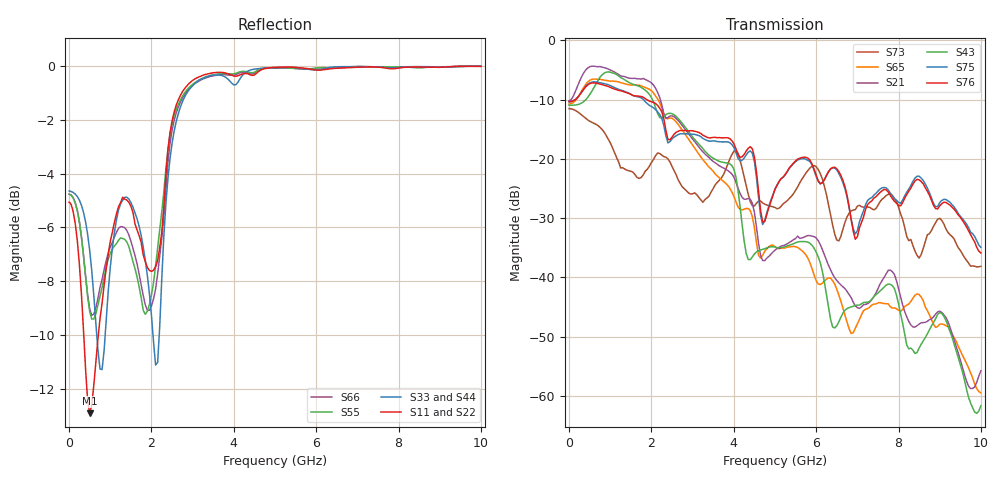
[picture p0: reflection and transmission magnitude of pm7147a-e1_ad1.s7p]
# GHz S DB R 50
! S-Parameters data
! Freq  dbS11  angS11  dbS12  angS12  dbS13  angS13  dbS14  angS14
!  dbS15  angS15  dbS16  angS16  dbS17  angS17  dbS21  angS21
!  dbS22  angS22  dbS23  angS23  dbS24  angS24  dbS25  angS25
!  dbS26  angS26  dbS27  angS27  dbS31  angS31  dbS32  angS32
!  dbS33  angS33  dbS34  angS34  dbS35  angS35  dbS36  angS36
!  dbS37  angS37  dbS41  angS41  dbS42  angS42  dbS43  angS43
!  dbS44  angS44  dbS45  angS45  dbS46  angS46  dbS47  angS47
!  dbS51  angS51  dbS52  angS52  dbS53  angS53  dbS54  angS54
!  dbS55  angS55  dbS56  angS56  dbS57  angS57  dbS61  angS61
!  dbS62  angS62  dbS63  angS63  dbS64  angS64  dbS65  angS65
!  dbS66  angS66  dbS67  angS67  dbS71  angS71  dbS72  angS72
!  dbS73  angS73  dbS74  angS74  dbS75  angS75  dbS76  angS76
!  dbS77  angS77
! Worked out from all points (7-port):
!   279 points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, 1 Hz to 10 GHz, reference 50 ohm
!   strongest paths, dB at 1 Hz, 7.943 MHz, 3.05 GHz, 6.55 GHz, 10 GHz:
!     S76: -10.3, -10.3, -15.3, -22.2, -35.9
!     S75: -10.3, -10.3, -15.9, -22.5, -34.9
!     S43: -10.9, -10.9, -16.7, -47.5, -61.7
!     S21: -10.2, -10.2, -17.1, -40.9, -55.8
!     S65: -10.7, -10.7, -18.2, -43.0, -59.5
!     S73: -11.5, -11.5, -25.7, -33.8, -38.1
!   lowest |S11| = -12.9 dB at 500 MHz (marker M1), VSWR 1.58, Z = 31.6 + j0.484 ohm
!   |S11| at or under -10 dB: 355.4 MHz to 709.4 MHz (354 MHz wide, 66.5 % of centre)
